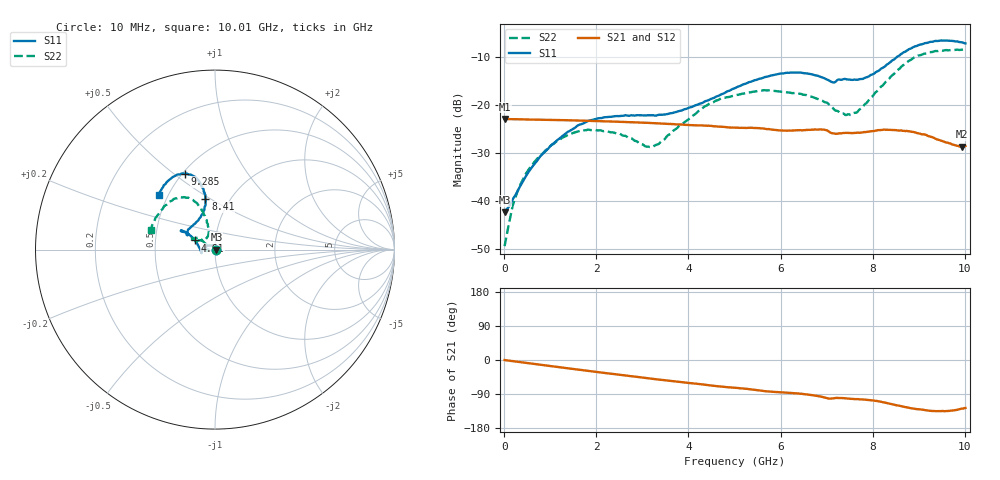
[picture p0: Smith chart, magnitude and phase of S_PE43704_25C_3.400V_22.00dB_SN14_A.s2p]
! Device ID: PE43704
! Dir: z:\PE43704\PE43704_Char_1_20130516\PE43704\AMB\3p400V\22p00dB
! Serial: 14
! Insertion: A
! Impedance: 50 ohm
! Temp: Amb
! VDD: 3.400V
! Attenuation Step: 22.00dB
! IDD: 1.141170e-01mA
#  Hz  S  RI  R  50
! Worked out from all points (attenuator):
!   401 points, 10 MHz to 10.01 GHz, reference 50 ohm
!   highest |S21| = -22.91 dB at 10 MHz (marker M1); lowest = -28.7 dB at 9.935 GHz (marker M2)
!   lowest |S11| = -42.3 dB at 10 MHz (marker M3), VSWR 1.02, Z = 50.8 + j0.0364 ohm
!   |S11| at or under -10 dB: start of sweep to 8.528 GHz
!   |S22| runs from -49.3 to -8.5 dB; largest |S21 - S12| = 0.00081
!   S11 on the Smith chart (normalised r, x): 10 MHz: 1.02, +0.00; 4.61 GHz: 0.80, +0.08; 8.41 GHz: 0.77, +0.47; 9.285 GHz: 0.52, +0.55; 10.01 GHz: 0.45, +0.33
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1e7  0.00771 0.000359  0.0715 -0.000272  0.0715 -0.000202  0.00339 0.000409
2.35e8  0.00558 0.00995  0.071 -0.0048  0.071 -0.00481  0.00183 0.0105
5.35e8  -0.00339 0.0201  0.07 -0.0107  0.07 -0.0107  -0.00634 0.0205
1.085e9  -0.0328 0.0235  0.0668 -0.0208  0.0668 -0.0208  -0.032 0.0237
1.685e9  -0.063 0.00727  0.0616 -0.0308  0.0616 -0.0308  -0.0541 0.00749
2.485e9  -0.0749 -0.0161  0.0523 -0.0418  0.0522 -0.0418  -0.05 -0.00686
3.11e9  -0.0767 -0.016  0.0438 -0.0485  0.0437 -0.0485  -0.0366 0.00471
3.36e9  -0.0785 -0.00981  0.0399 -0.0505  0.0399 -0.0504  -0.0372 0.0137
4.285e9  -0.0992 0.0327  0.0269 -0.0552  0.0269 -0.0552  -0.0735 0.0532
4.61e9  -0.1116 0.051  0.0217 -0.0559  0.0217 -0.0557  -0.0908 0.0645
5.01e9  -0.1311 0.0725  0.0168 -0.0558  0.0168 -0.0559  -0.1091 0.0625
5.96e9  -0.1821 0.1052  0.0048 -0.0545  0.00504 -0.0543  -0.128 0.0524
6.685e9  -0.1826 0.1003  -0.00282 -0.0556  -0.0027 -0.0553  -0.1133 0.0437
7.135e9  -0.1496 0.0845  -0.01 -0.0499  -0.00975 -0.0496  -0.0779 0.0507
7.535e9  -0.1284 0.13  -0.0112 -0.05  -0.0111 -0.0501  -0.0453 0.0645
7.86e9  -0.0879 0.1727  -0.0136 -0.0507  -0.0135 -0.0508  -0.0356 0.0979
8.36e9  -0.0526 0.2684  -0.0236 -0.0499  -0.0233 -0.0499  -0.0537 0.1808
8.41e9  -0.053 0.2819  -0.0247 -0.0492  -0.0244 -0.0494  -0.0605 0.1918
8.86e9  -0.0914 0.384  -0.0321 -0.0416  -0.0319 -0.0416  -0.1235 0.2769
9.285e9  -0.1669 0.4219  -0.0327 -0.0331  -0.0323 -0.0329  -0.2104 0.2862
9.935e9  -0.3021 0.3296  -0.0227 -0.029  -0.0233 -0.0288  -0.3474 0.1404
1.001e10  -0.3136 0.3044  -0.0224 -0.0302  -0.0221 -0.0298  -0.3568 0.111
